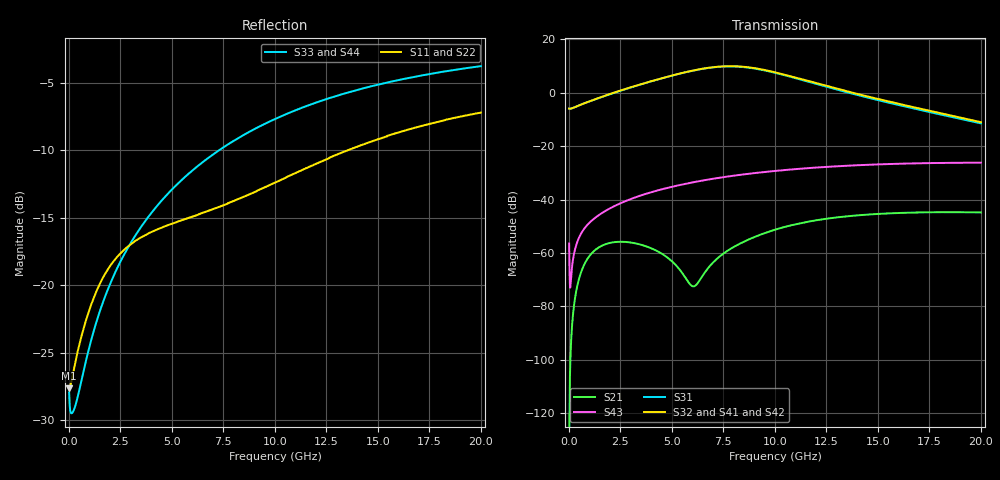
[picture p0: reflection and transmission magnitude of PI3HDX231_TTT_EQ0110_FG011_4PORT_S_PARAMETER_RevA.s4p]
! NPort=4 DATA=2000 NOISE=0 GROUPDELAY=0 COMPLEX_DATAFORMAT=POLAR
! NumOfBlock=1 NumOfParam=0
! .MODEL Smodel S TSTONEFILE=PI3HDX231_TTT_EQ0110_FG011_4PORT_S_PARAMETER_RevA.s4p TYPE=S
!  -- The above .MODEL line can be used for the S element in the netlist.
! The s parameter is extracted from the linear redriver, it is not bi-directional; only s(4,1)s(4,2) and s(3,1)s(3,2)
! should be the insertion loss
!Port definition:
!Port1 = input+
!Port2 = input-
!Port3 = output+
!Port4 = output-
# Hz S MA R  50
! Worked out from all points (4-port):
!   2000 points, 10 MHz to 20 GHz, reference 50 ohm
!   strongest paths, dB at 10 MHz, 5.01 GHz, 10.01 GHz, 15.01 GHz, 20 GHz:
!     S32: -5.9, 6.4, 7.6, -2.4, -11.0
!     S41: -5.9, 6.5, 7.6, -2.4, -11.2
!     S42: -5.9, 6.5, 7.6, -2.6, -11.2
!     S31: -5.9, 6.4, 7.5, -2.8, -11.5
!     S43: -56.5, -35.2, -29.3, -26.9, -26.2
!     S21: -134.8, -63.2, -51.3, -45.4, -44.9
!   lowest |S11| = -27.6 dB at 10 MHz (marker M1), VSWR 1.09, Z = 46 - j0.0776 ohm
!   |S11| at or under -10 dB: start of sweep to 13.55 GHz
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1e7  0.04152 -178.8  1.825e-07 -13.9  0 0.0  0 0.0
     1.825e-07 -14.0  0.04152 -178.8  0 0.0  0 0.0
     0.5042 -0.4  0.5042 179.6  0.04012 -3.2  0.0015 -70.3
     0.5042 179.6  0.5042 -0.4  0.0015 -70.3  0.04012 -3.2
4.97e9  0.1686 -140.1  0.0007118 -13.3  5.429e-10 -169.1  2.888e-10 -145.1
        0.0007142 -13.2  0.1686 -140.2  2.79e-10 -144.9  5.65e-10 -169.0
        2.074 -51.6  2.079 127.9  0.2248 -102.4  0.01722 61.8
        2.086 127.8  2.094 -50.8  0.01718 61.7  0.2248 -102.4
6.93e9  0.1904 -136.0  0.0006228 98.5  4.316e-09 127.8  2.02e-09 -177.3
        0.000621 97.5  0.1901 -136.3  1.959e-09 -176.1  4.509e-09 126.8
        2.961 -110.1  2.979 69.6  0.3023 -107.9  0.02432 50.3
        2.985 69.4  2.998 -109.1  0.02423 50.2  0.3024 -107.9
8.61e9  0.2144 -132.1  0.001715 95.3  1.436e-08 73.5  9.321e-09 139.7
        0.001703 94.8  0.2136 -132.3  9.124e-09 141.3  1.493e-08 71.6
        2.982 -169.8  3.022 9.9  0.3641 -112.2  0.03007 39.6
        3.024 9.5  3.023 -168.8  0.02995 39.6  0.3643 -112.3
1.09e10  0.2582 -128.6  0.003389 74.6  4.233e-08 12.9  3.585e-08 66.7
         0.003365 74.2  0.2567 -128.8  3.547e-08 68.5  4.322e-08 10.3
         1.918 119.7  1.971 -61.0  0.4409 -117.8  0.03692 24.6
         1.967 -61.5  1.948 120.9  0.03679 24.8  0.441 -117.8
1.389e10  0.3231 -128.6  0.005043 44.0  1.162e-07 -51.3  9.702e-08 -13.4
          0.005004 43.8  0.321 -128.6  9.711e-08 -11.7  1.167e-07 -53.8
          0.9306 55.9  0.9734 -126.0  0.5253 -124.3  0.04368 5.1
          0.9662 -126.5  0.9499 57.5  0.04361 5.4  0.5251 -124.3
2e10  0.4355 -135.6  0.005768 -4.5  3.721e-07 -159.8  2.761e-07 -134.9
      0.005721 -4.6  0.4338 -135.4  2.792e-07 -134.0  3.671e-07 -161.8
      0.2665 -39.5  0.2805 134.6  0.6464 -135.0  0.04883 -32.3
      0.2767 134.6  0.2763 -37.9  0.04893 -32.0  0.6461 -135.0
